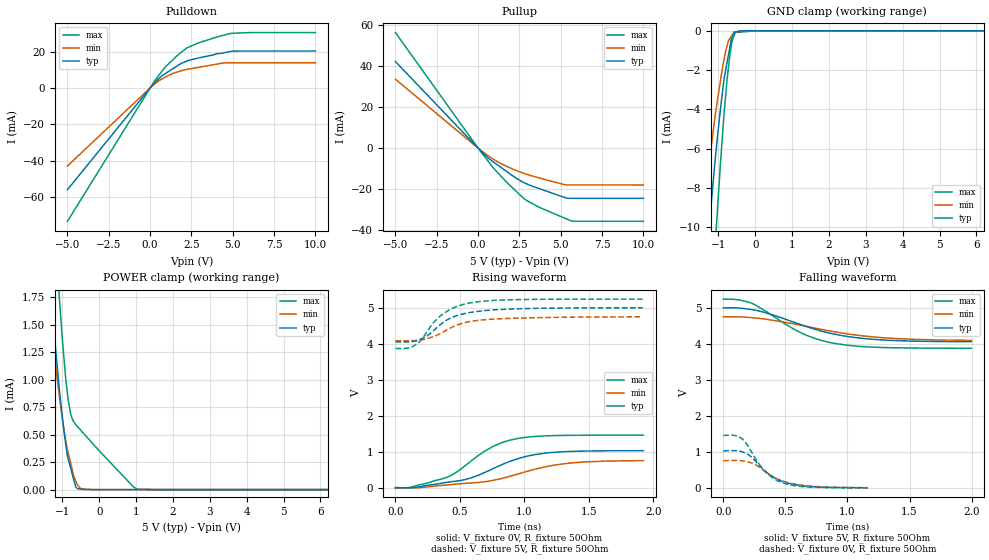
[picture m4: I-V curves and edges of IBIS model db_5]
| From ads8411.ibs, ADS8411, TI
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|   db_5 Model
[Model]   db_5
Model_type   3-state
Polarity   Non-Inverting
Vmeas = 2.5
Vref = 2.5
Cref = 20pF
Rref = 50
|   typ   min   max
|   (nom PVT)   (fast PVT)   (slow PVT)
|C_comp from frequency sweep method (F=1MHz)
|C_comp   3.282e-12   3.237e-12   3.331e-12
|ON state : BUFFER OUTPUT TURNED HIGH
|C_comp   3.282e-12   3.237e-12   3.331e-12
|OFF state: BUFFER IN HIGH IMPEDANCE
|C_comp   3.268e-12   3.233e-12   3.305e-12
|C_comp from LC tank measurement(L=1nH)
|Resonant Frequency(Hz)   3.030e+09   3.060e+09   2.990e+09
C_comp   2.762e-12   2.708e-12   2.836e-12
|ON state : BUFFER OUTPUT TURNED HIGH
|Resonant Frequency(Hz)   3.040e+09   3.070e+09   3.010e+09
|C_comp   2.744e-12   2.690e-12   2.799e-12
|OFF state: BUFFER IN HIGH IMPEDANCE
|Resonant Frequency(Hz)   3.030e+09   3.060e+09   2.990e+09
|C_comp   2.762e-12   2.708e-12   2.836e-12
| Where nom  PVT is Nominal Process, 5V, 40C
|   Fast PVT is Strong Process,  5.25V, -40C
|   Slow PVT is Weak Process,   4.75V, 100C
[Voltage Range]   5   4.75   5.25
|Ambient Temperature   25   85   -40
|Junction Temperature
[Temperature Range]   40   100   -40
[Pullup Reference]   5   4.75   5.25
[Pulldown Reference]   0   0   0
[Power Clamp Reference]   5   4.75   5.25
[GND Clamp Reference]   0   0   0
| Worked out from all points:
|   slope of the pulldown table from 0 to 0.75 V, typ, clamps not added: 108 ohm
|   slope of the pullup table from 0 to 0.75 V, typ, clamps not added: 131 ohm
|   GND clamp passes 1 mA (typ) near -0.70 V on its own axis
|   POWER clamp passes 1 mA (typ) near -1.11 V on its own axis
|   falling waveform, V_fixture 5V, R_fixture 50Ohm: 20-80 % time 543ps typ, 653ps min, 428ps max; typ from 5 V to 4.06 V
|   rising waveform, V_fixture 0V, R_fixture 50Ohm: 20-80 % time 458ps typ, 547ps min, 371ps max; typ from 0 V to 1.03 V
|   rising waveform, V_fixture 5V, R_fixture 50Ohm: 20-80 % time 250ps typ, 264ps min, 224ps max; typ from 4.05 V to 5 V
|   falling waveform, V_fixture 0V, R_fixture 50Ohm: 20-80 % time 218ps typ, 236ps min, 193ps max; typ from 1.03 V to 0.004 V
[Pulldown]
|   Voltage   I(typ)   I(min)   I(max)
-5V       -56.07mA   -43.01mA   -73.51mA
252mV     2.669mA    2.026mA    3.652mA
700mV     6.638mA    4.914mA    9.138mA
924mV     7.959mA    6.012mA    11.61mA
1.825V    13.27mA    9.335mA    19.33mA
2.226V    14.86mA    10.26mA    22.11mA
2.94V     16.57mA    11.41mA    24.93mA
4.052V    18.96mA    13.2mA     28.12mA
4.403V    19.29mA    13.74mA    29.01mA
4.956V    20.3mA     13.89mA    30.18mA
10V       20.41mA    13.94mA    30.56mA
[GND Clamp]
|   Voltage   I(typ)   I(min)   I(max)
-5V       -1.352A    -1.001A    -1.995A
-1.533V   -18.92mA   -11.53mA   -26.89mA
-1.306V   -11.12mA   -7.6mA     -18.27mA
-1.176V   -8.416mA   -5.646mA   -13.85mA
-1.05V    -5.864mA   -3.842mA   -9.845mA
-865mV    -2.749mA   -1.616mA   -4.724mA
-766.5mV  -1.639mA   -785.7uA   -2.538mA
-687.7mV  -834.8uA   -391.1uA   -1.233mA
-640.5mV  -352.6uA   -258.8uA   -666uA
-570mV    -99.93uA   -61.4uA    -224.7uA
-84.44fV  0A         0A         0A
10V       0A         0A         0A
[Pullup]
|   Voltage   I(typ)   I(min)   I(max)
-5V       42.36mA    33.71mA    56.54mA
115.6fV   -8.124pA   -3.453pA   -3.426uA
475mV     -3.799mA   -2.975mA   -4.998mA
924mV     -6.747mA   -5.422mA   -9.72mA
1.596V    -10.65mA   -8.424mA   -15.56mA
2.27V     -14.56mA   -10.86mA   -20.86mA
2.767V    -16.82mA   -12.35mA   -24.63mA
3.602V    -19.53mA   -14.39mA   -28.57mA
5.18V     -24mA      -17.77mA   -34.06mA
5.405V    -24.56mA   -18mA      -34.83mA
5.696V    -24.56mA   -18mA      -35.81mA
10V       -24.56mA   -18.01mA   -35.81mA
[POWER Clamp]
|   Voltage   I(typ)   I(min)   I(max)
-5V       1.348A     997.9mA    1.981A
-1.517V   2.821mA    3.859mA    4.946mA
-1.31V    1.741mA    1.539mA    3.008mA
-1.085V   913.2uA    850.4uA    1.751mA
-997.5mV  646uA      630.8uA    1.345mA
-913.5mV  421.6uA    452.9uA    1.019mA
-845.2mV  278.9uA    336.7uA    818.2uA
-714mV    115.6uA    151.7uA    626.8uA
-595mV    8.714uA    43.23uA    574.2uA
-190mV    0A         0A         423.2uA
1.04V     0A         0A         2.581uA
10V       0A         0A         0A
[Ramp]
R_load = 50
|   typ   min   max
dV/dt_r   0.620278/4.56679e-10   0.456847/5.48021e-10   0.87779/3.69716e-10
dV/dt_f   0.568773/5.44165e-10   0.399467/6.69082e-10   0.822011/4.29907e-10
[Falling Waveform]
V_fixture = 5V
V_fixture_min = 4.75V
V_fixture_max = 5.25V
R_fixture = 50Ohm
|   Time   V(typ)   V(min)   V(max)
0s        5V         4.75V      5.239V
109ps     4.994V     4.748V     5.225V
228ps     4.948V     4.724V     5.125V
321ps     4.882V     4.693V     4.946V
602ps     4.557V     4.529V     4.344V
740ps     4.401V     4.434V     4.145V
866ps     4.288V     4.35V      4.031V
1.088ns   4.162V     4.233V     3.93V
1.281ns   4.106V     4.169V     3.897V
1.998ns   4.056V     4.094V     3.873V
[Rising Waveform]
V_fixture = 0V
V_fixture_min = 0V
V_fixture_max = 0V
R_fixture = 50Ohm
|   Time   V(typ)   V(min)   V(max)
0s        1.868nV    2.766nV    1.738nV
119ps     3.745mV    1.338mV    18.7mV
401ps     154.8mV    79.69mV    294.7mV
471ps     186.6mV    103.7mV    430.2mV
581ps     270.2mV    134.3mV    727.9mV
755ps     530.5mV    206.3mV    1.146V
946ps     806.3mV    380.9mV    1.369V
1.079ns   921.2mV    514.4mV    1.426V
1.315ns   1.005V     672.3mV    1.456V
1.923ns   1.032V     756.5mV    1.463V
[Rising Waveform]
V_fixture = 5V
V_fixture_min = 4.75V
V_fixture_max = 5.25V
R_fixture = 50Ohm
|   Time   V(typ)   V(min)   V(max)
0s        4.052V     4.084V     3.869V
100ps     4.052V     4.082V     3.882V
146ps     4.072V     4.086V     3.95V
191ps     4.121V     4.101V     4.073V
250ps     4.231V     4.146V     4.362V
357ps     4.557V     4.298V     4.796V
442ps     4.736V     4.464V     4.983V
573ps     4.865V     4.615V     5.129V
984ps     4.974V     4.715V     5.228V
1.917ns   4.999V     4.748V     5.239V
[Falling Waveform]
V_fixture = 0V
V_fixture_min = 0V
V_fixture_max = 0V
R_fixture = 50Ohm
|   Time   V(typ)   V(min)   V(max)
0s        1.034V     761.5mV    1.463V
93ps      1.034V     763.3mV    1.454V
150ps     1.004V     753.2mV    1.366V
188ps     950.4mV    732.6mV    1.223V
228ps     852.7mV    690.8mV    989.7mV
323ps     509.1mV    489.8mV    507.3mV
391ps     324.1mV    328.9mV    292.6mV
466ps     191.4mV    206.3mV    155.5mV
690ps     41.73mV    53.66mV    22.08mV
1.164ns   3.846mV    6.679mV    1.388mV
